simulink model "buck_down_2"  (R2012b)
settings: Solver=ode45  StartTime=0.0  StopTime=10.0  RelTol=1e-3
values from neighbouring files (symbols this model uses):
  C = 100e-6    (= 0.0001)    [boost_up1.m]    (also in buck_boost1.m = 0.0002; buck_boost2.m = 0.0002; buck_down1.m; buck_down2.m)
  kd = 0.5    [buck_down2.m]
  ki = 50    [buck_down2.m]
  kr = 200    [buck_down2.m]
  L = 0.001    [boost_up1.m]    (also in buck_boost1.m; buck_boost2.m; buck_down1.m; buck_down2.m)
  R = 5    [boost_up1.m]    (also in buck_boost1.m; buck_boost2.m; buck_down1.m = 2*Rmax,; buck_down2.m = 0.1*Rmax,)
  T = 1/f0    (= 5e-05)    [boost_up1.m]    (also in buck_boost1.m; buck_boost2.m; buck_down1.m; buck_down2.m)
  Ui = 5    [boost_up1.m]    (also in buck_boost1.m; buck_boost2.m; buck_down1.m; buck_down2.m)
  Usoll = 2    [buck_down2.m]
libraries: simulink x1

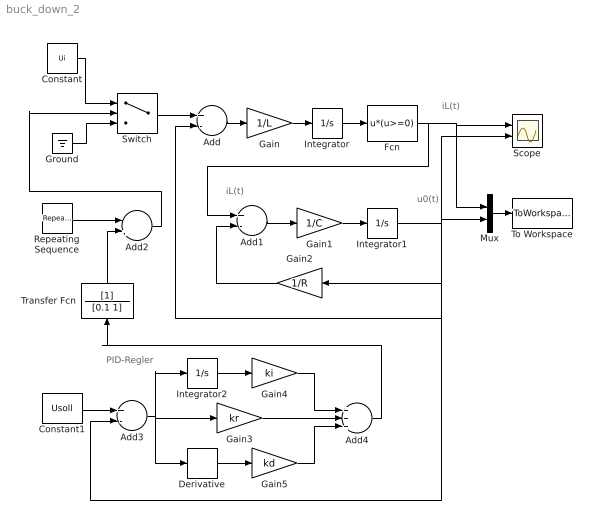
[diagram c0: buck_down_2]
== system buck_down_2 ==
  note: PID-Regler
  note: iL(t)
  note: u0(t)
  note: iL(t)
  Add : Sum  Inputs=+-
  Add1 : Sum  Inputs=+-
  Add2 : Sum  Inputs=-+
  Add3 : Sum  Inputs=+-
  Add4 : Sum  Inputs=+++
  Constant : Constant  Value=Ui
  Constant1 : Constant  Value=Usoll
  Derivative : Derivative
  Fcn : Fcn  Expr=u*(u>=0)
  Gain : Gain  Gain=1/L
  Gain1 : Gain  Gain=1/C
  Gain2 : Gain  Gain=1/R
  Gain3 : Gain  Gain=kr
  Gain4 : Gain  Gain=ki
  Gain5 : Gain  Gain=kd
  Ground : Ground
  Integrator : Integrator
  Integrator1 : Integrator
  Integrator2 : Integrator
  Mux : Mux  Inputs=2
  Repeating Sequence : simulink/Sources/Repeating Sequence  rep_seq_t=[0 T]  rep_seq_y=[0 1]
  Scope : Scope  NumInputPorts=2
  Switch : Switch  Criteria=u2 > Threshold  SampleTime=0
  To Workspace : ToWorkspace  VariableName=y  SampleTime=-1  SaveFormat=Structure With Time
  Transfer Fcn : TransferFcn  Denominator=[0.1 1]
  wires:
  Add/1 -> Gain/1
  Gain/1 -> Integrator/1
  Gain1/1 -> Integrator1/1
  Add1/1 -> Gain1/1
  Gain2/1 -> Add1/2
  Ground/1 -> Switch/3
  Constant/1 -> Switch/1
  Switch/1 -> Add/1
  Integrator/1 -> Fcn/1
  Fcn/1 -> Add1/1, Mux/1, Scope/1
  Mux/1 -> To Workspace/1
  Repeating Sequence/1 -> Add2/1
  Constant1/1 -> Add3/1
  Add3/1 -> Derivative/1, Integrator2/1, Gain3/1
  Gain3/1 -> Add4/2
  Integrator2/1 -> Gain4/1
  Gain4/1 -> Add4/1
  Gain5/1 -> Add4/3
  Derivative/1 -> Gain5/1
  Add2/1 -> Switch/2
  Integrator1/1 -> Mux/2, Scope/2, Gain2/1, Add3/2, Add/2
  Add4/1 -> Transfer Fcn/1
  Transfer Fcn/1 -> Add2/2
